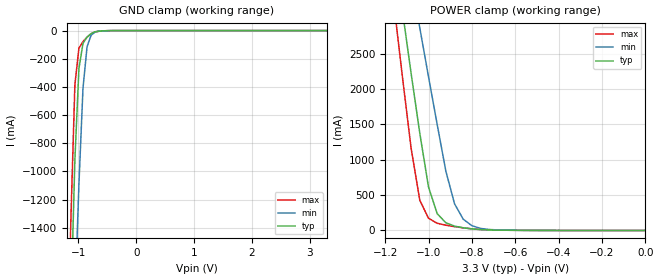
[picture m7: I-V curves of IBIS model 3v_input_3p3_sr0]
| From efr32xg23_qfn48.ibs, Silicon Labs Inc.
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|   Model 3v_input_3p3_sr0
[Model]  3v_input_3p3_sr0
Model_type Input
C_comp   1.6300pF   1.4000pF   2.7000pF
[Temperature Range]   25.0000   0.1250k   -40.0000
[Pullup Reference]   3.3000V   3.0000V   3.6000V
[Pulldown Reference]   0.0V   0.0V   0.0V
[POWER Clamp Reference]   3.3000V   3.0000V   3.6000V
[GND Clamp Reference]   0.0V   0.0V   0.0V
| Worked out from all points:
|   GND clamp passes 1 mA (typ) near -0.52 V on its own axis
|   POWER clamp passes 1 mA (typ) near -0.53 V on its own axis
[GND_clamp]
|Voltage   I(typ)   I(min)   I(max)
-3.3V     -36.82A    -34.37A    -38.92A
-1.2V     -3.169A    -3.961A    -2.635A
-1.13V    -1.976A    -2.875A    -1.354A
-1.06V    -919.5mA   -1.925A    -386.3mA
-990mV    -269.8mA   -1.092A    -124.2mA
-920mV    -91.07mA   -411.1mA   -78.21mA
-850mV    -46.3mA    -116.2mA   -47.38mA
-780mV    -21.47mA   -33.46mA   -23mA
-710mV    -8.335mA   -10.37mA   -9.191mA
-430mV    -188uA     -421.9uA   -101.6uA
3.3V      1.131nA    22.57uA    998.8pA
[POWER_clamp]
|Voltage   I(typ)   I(min)   I(max)
-3.28V    55.25A     49.02A     61.14A
-1.16V    4.026A     5.102A     3.218A
-1.12V    3.102A     4.316A     2.168A
-1.08V    2.218A     3.57A      1.158A
-1.04V    1.373A     2.863A     426mA
-1V       614.4mA    2.175A     173.2mA
-960mV    237.7mA    1.5A       101.5mA
-920mV    109.2mA    839mA      74.96mA
-880mV    61.4mA     377.7mA    54.07mA
-840mV    37.94mA    159.6mA    37.09mA
-720mV    7.455mA    13.75mA    7.89mA
0V        1.131nA    10.99nA    1.2nA
